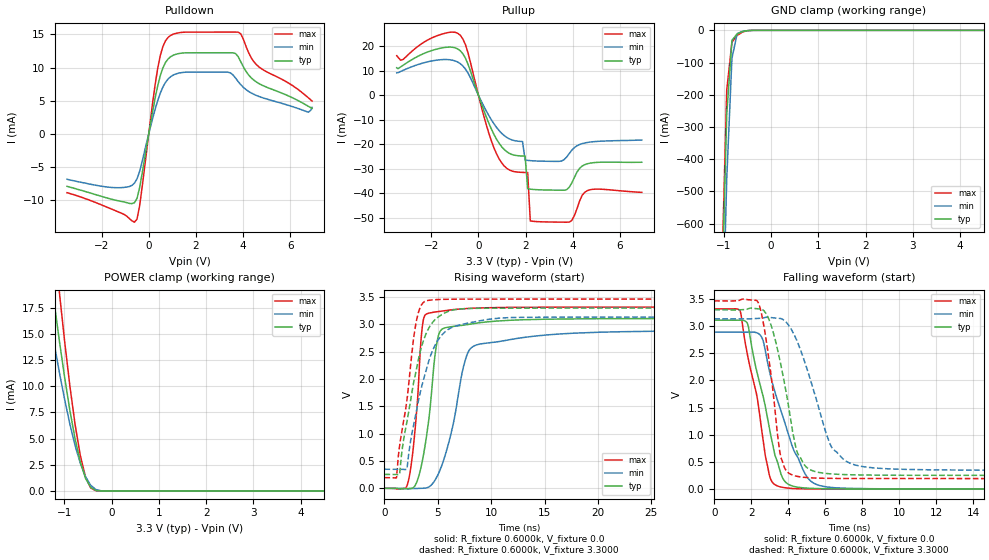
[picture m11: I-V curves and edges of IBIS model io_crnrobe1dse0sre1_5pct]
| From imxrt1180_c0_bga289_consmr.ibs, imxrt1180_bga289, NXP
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[Model]  io_crnrobe1dse0sre1_5pct
|   Model io_crnrobe1dse0sre1_5pct
| This model was characterised for following simulation conditions:
| External (pad) voltage:
|   - Typ: 3.3V,   - Min: 3.135V,   - Max: 3.465V
| Library cells for typ/min/max conditions are connected as defined below:
|  PAD_IO - External Pad
|  ipp_do - Core Input
|  ipp_obe - Output Buffer Enable
|  ASRCN3V3[3] - NC
|  ASRCN3V3[4] - NC
|  ASRCP3V3[4] - NC
|  REFAPBIAS3V3 - gnde
|  REFBAMPL3V3 - vdd1v8
|  REFCAMPH3V3 - vdd1v8
|  REFDNBIAS3V3 - vdd1v8
|  REFH3V3 - REFH3V3
|  REFL3V3 - REFL3V3
|  gnde - gnde
|  ipp_dse - gnde
|  ipp_ina235_3v - NC
|  ipp_ina40_3v - NC
|  ipp_ina_mux - NC
|  ipp_ind - NC
|  ipp_ind_1p8v - NC
|  ipp_ind_3v - NC
|  ipp_sre - vdd
|  vdd - vdd
|  vdd1v8 - vdd1v8
|  vdda - vdde3v3
|  vdde3v3 - vdde3v3
| All other pins connected to ground
Model_type I/O
Polarity   Non-Inverting
Enable   Active-High
Vinl =   0.9900V
Vinh =   2.3100V
Vmeas =  1.6500V
Cref =   15.0000pF
Rref =   0.6000k
Vref =   0.0V
C_comp   4.0038pF   3.8208pF   4.1241pF
|C_comp_pullup   0.5150pF   0.5903pF   0.4959pF
|C_comp_pulldown   2.0815pF   2.1811pF   1.8613pF
[Model Spec]
| variable   typ   min   max
Vinh   2.3100V   NA   NA
Vinl   0.9900V   NA   NA
Vref   0.0V   0.0V   0.0V
Cref   15.0000pF   15.0000pF   15.0000pF
Rref   0.6000k   0.6000k   0.6000k
[Receiver Thresholds]
Vcross_high  =   0.0V
Vcross_low  =   0.0V
Vdiff_ac  =   0.0V
Vdiff_dc  =   0.0V
Tdiffslew_ac  =   0.0S
[Temperature Range]   25.0000   0.1250k   -40.0000
[Voltage Range]   3.3000V   3.1350V   3.4650V
[Pullup Reference]   3.3000V   3.1350V   3.4650V
[Pulldown Reference]   0.0V   0.0V   0.0V
[POWER Clamp Reference]   3.3000V   3.1350V   3.4650V
[GND Clamp Reference]   0.0V   0.0V   0.0V
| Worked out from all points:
|   slope of the pulldown table from 0 to 0.495 V, typ, clamps not added: 56 ohm
|   slope of the pullup table from 0 to 0.495 V, typ, clamps not added: 39.3 ohm
|   GND clamp passes 1 mA (typ) near -0.50 V on its own axis
|   POWER clamp passes 1 mA (typ) near -0.52 V on its own axis
|   rising waveform, R_fixture 0.6000k, V_fixture 0.0: 20-80 % time 1.1ns typ, 1.87ns min, 744ps max; typ from 0 V to 3.11 V
|   rising waveform, R_fixture 0.6000k, V_fixture 3.3000: 20-80 % time 1.85ns typ, 2.15ns min, 1.31ns max; typ from 0.254 V to 3.3 V
|   falling waveform, R_fixture 0.6000k, V_fixture 0.0: 20-80 % time 1.19ns typ, 1.63ns min, 1.04ns max; typ from 3.11 V to 0 V
|   falling waveform, R_fixture 0.6000k, V_fixture 3.3000: 20-80 % time 1.01ns typ, 1.53ns min, 701ps max; typ from 3.3 V to 0.254 V
[Pulldown]
|Voltage   I(typ)   I(min)   I(max)
-3.465V   -7.9mA     -6.83mA    -8.86mA
-1.265V   -10.1mA    -8.106mA   -11.79mA
-495mV    -9.702mA   -6.762mA   -12.83mA
-385mV    -8.098mA   -5.646mA   -10.83mA
385mV     7.308mA    5.061mA    9.964mA
605mV     9.988mA    7.101mA    13.21mA
1.045V    11.88mA    8.891mA    15.06mA
3.355V    12.25mA    9.322mA    15.36mA
3.795V    11.65mA    7.905mA    15.35mA
4.565V    7.843mA    5.809mA    10.46mA
6.765V    4.186mA    3.281mA    5.474mA
6.93V     3.841mA    4.012mA    4.963mA
[Pullup]
|Voltage   I(typ)   I(min)   I(max)
-3.465V   11.16mA    9.087mA    16.08mA
-1.76V    18.78mA    14.27mA    24.18mA
-770mV    18.07mA    12.84mA    24.39mA
-440mV    12.59mA    8.971mA    17.18mA
770mV     -17.95mA   -13.16mA   -23.93mA
1.87V     -24.79mA   -18.89mA   -31.45mA
1.98V     -24.83mA   -26.37mA   -31.49mA
2.09V     -38.08mA   -26.55mA   -31.51mA
2.2V      -38.26mA   -26.66mA   -51.22mA
3.85V     -37.51mA   -23.82mA   -51.7mA
4.73V     -27.69mA   -19.1mA    -38.53mA
6.93V     -27.31mA   -18.28mA   -39.57mA
[GND_clamp]
|Voltage   I(typ)   I(min)   I(max)
-3.465V   -18.65A    -18.54A    -19.59A
-1.045V   -856.4mA   -1.07A     -789.2mA
-935mV    -262.9mA   -462.2mA   -186.4mA
-825mV    -31.14mA   -87.01mA   -37.16mA
-715mV    -11.21mA   -10.51mA   -15.88mA
-605mV    -3.859mA   -3.519mA   -5.394mA
-385mV    -79.67uA   -219.6uA   -43.93uA
6.93V     0A         0A         0A
[POWER_clamp]
|Voltage   I(typ)   I(min)   I(max)
-3.465V   98.91mA    78.43mA    126mA
-1.43V    25.78mA    19.9mA     34.19mA
-1.32V    21.78mA    16.89mA    28.92mA
-1.21V    17.92mA    14mA       23.79mA
-1.1V     14.24mA    11.26mA    18.86mA
-880mV    7.673mA    6.373mA    9.998mA
-770mV    4.965mA    4.333mA    6.33mA
-660mV    2.777mA    2.644mA    3.379mA
-550mV    1.212mA    1.363mA    1.332mA
-440mV    333.5uA    531.5uA    282.6uA
-330mV    37.61uA    130.9uA    15.04uA
6.93V     0A         0A         0A
[Ramp]
| variable   typ   min   max
dV/dt_r  1.8668/1.1025n   1.7338/1.8703n   1.9910/0.7441n
dV/dt_f  1.8274/1.0132n   1.6719/1.5287n   1.9622/0.7015n
R_load = 0.6000k
[Rising Waveform]
R_fixture= 0.6000k
V_fixture= 0.0
V_fixture_min= 0.0
V_fixture_max= 0.0
|time   V(typ)   V(min)   V(max)
0s        139.9nV    3.48uV     63.01nV
2.202ns   -5.191mV   -12.23mV   105.3mV
2.877ns   52.66mV    -3.184mV   1.096V
3.543ns   496.4mV    -436.1uV   2.958V
4.101ns   1.182V     18.58mV    3.204V
4.722ns   2.422V     144.2mV    3.228V
5.171ns   2.86V      319.3mV    3.237V
7.588ns   2.993V     2.362V     3.291V
8.716ns   3.027V     2.631V     3.301V
60ns      3.111V     2.89V      3.318V
[Rising Waveform]
R_fixture= 0.6000k
V_fixture= 3.3000
V_fixture_min= 3.1350
V_fixture_max= 3.4650
|time   V(typ)   V(min)   V(max)
0s        254.3mV    348.5mV    194.7mV
1.119ns   253.6mV    348.4mV    192.2mV
1.42ns    265.1mV    347.9mV    784.3mV
2.098ns   1.216V     352.6mV    1.607V
2.935ns   2.123V     1.355V     3.006V
3.883ns   2.825V     2.148V     3.432V
4.842ns   3.107V     2.658V     3.455V
5.888ns   3.232V     2.899V     3.462V
10.82ns   3.298V     3.117V     3.465V
60ns      3.3V       3.135V     3.465V
[Falling Waveform]
R_fixture= 0.6000k
V_fixture= 0.0
V_fixture_min= 0.0
V_fixture_max= 0.0
|time   V(typ)   V(min)   V(max)
0s        3.111V     2.89V      3.318V
1.39ns    3.112V     2.89V      3.289V
1.809ns   3.041V     2.888V     2.455V
2.317ns   2.147V     2.877V     1.701V
2.561ns   1.825V     2.802V     1.108V
2.997ns   1.096V     2.16V      241.4mV
3.79ns    157mV      1.256V     27.51mV
5.061ns   17.96mV    206.6mV    4.007mV
6.541ns   5.089mV    25.87mV    695.4uV
60ns      2.332uV    4.359uV    1.975uV
[Falling Waveform]
R_fixture= 0.6000k
V_fixture= 3.3000
V_fixture_min= 3.1350
V_fixture_max= 3.4650
|time   V(typ)   V(min)   V(max)
0s        3.3V       3.135V     3.465V
2.367ns   3.319V     3.14V      3.443V
2.848ns   3.205V     3.164V     2.662V
3.59ns    2.313V     3.141V     611.1mV
4.376ns   831.5mV    2.807V     244.5mV
4.659ns   582.5mV    2.572V     225.5mV
5.18ns    359.7mV    2.042V     209mV
6.347ns   280.1mV    776mV      197.9mV
8.384ns   259.1mV    399.7mV    194.9mV
60ns      254.3mV    348.5mV    194.7mV
